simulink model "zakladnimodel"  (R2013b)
settings: Solver=FixedStepDiscrete  StartTime=0.0  StopTime=132.0  FixedStep=1  RelTol=1e-3

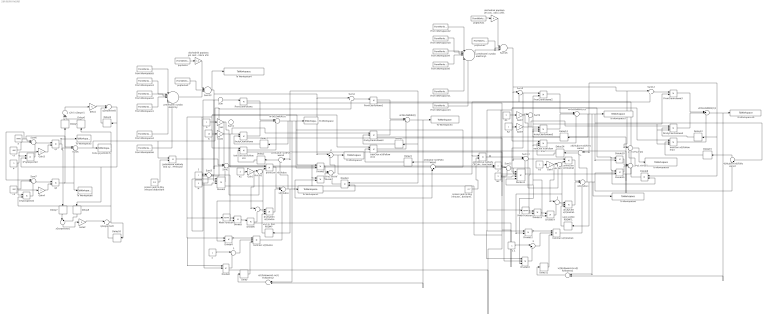
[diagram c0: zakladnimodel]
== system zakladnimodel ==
  " " : Sum  Inputs=|++
  " x1(t-1) POC PODM?" : Delay  DelayLength=1  InitialCondition=0
  " x1(t-1) POC PODM?1" : Delay  DelayLength=1  InitialCondition=0
  " x(t)Followera1+x(t)Followera1" : Sum  Inputs=|++
  " x(t)Followera1+x(t)Followera2" : Sum  Inputs=|++
   x(t)Vudce+x(t)Followera{1..4} (4 alike) : Sum  Inputs=|++
  " x2t-1-x2expt-1" : Sum  Inputs=|+-
  " 1" : Sum  Inputs=|+-
  " 2" : Sum  Inputs=|++
  " 2A+2K1" : Sum  Inputs=|++
  " 2A+2K2" : Sum  Inputs=|++
  " 3" : Sum  Inputs=|+-
  " A*x1+A*xV" : Sum  Inputs=|+++
  " A*x1+A*xV1" : Sum  Inputs=|+++
  " P" : Sum  Inputs=|+-
  " prednostni vyroba elektriny" : Sum  Inputs=|+++++++
  " prednostni vyroba elektriny1" : Sum  Inputs=|+++++++
  " q1expectedt" : Sum  Inputs=|++
  " q2expectedt " : Sum  Inputs=|++
  " x(t)Vudce" : Sum  Inputs=|++-
  " x(t)Vudce1" : Sum  Inputs=|++-
  " x2expectedt1" : Sum  Inputs=|+-
  " xFOLLOWER1(t)" : Sum  Inputs=|++-
  " xFOLLOWER1(t)1" : Sum  Inputs=|++-
  " xFOLLOWER2(t)" : Sum  Inputs=|++-
  " xFOLLOWER2(t)1" : Sum  Inputs=|++-
  1 : Constant
  "1 " : Constant
  1 1 : Constant
  2 : Constant
  A : Constant
  A1 : Constant
  "Cena je jednotk.N " : ToWorkspace  VariableName=Puhli  SampleTime=-1  SaveFormat=Timeseries
  Delay{,1..15} (16 alike) : Delay  DelayLength=1  InitialCondition=0
  Divide{1..2,5,7,9..10,13,15} (8 alike) : Product  Inputs=**
  Divide11 : Product  Inputs=***/
  Divide{4,6,12,14} (4 alike) : Product  Inputs=*/
  Divide16 : Product  Inputs=**/
  Divide3 : Product  Inputs=***/
  Divide8 : Product  Inputs=**/
  DruhyClenFollowa{,1..3} (4 alike) : Product  Inputs=**/
  From Workspace1 : FromWorkspace  VariableName=FVE  SampleTime=0
  From Workspace10 : FromWorkspace  VariableName=JE  SampleTime=0
  From Workspace11 : FromWorkspace  VariableName=ostatni  SampleTime=0
  From Workspace12 : FromWorkspace  VariableName=bioplyn  SampleTime=0
  From Workspace13 : FromWorkspace  VariableName=biomasa  SampleTime=0
  From Workspace2 : FromWorkspace  VariableName=VE  SampleTime=0
  From Workspace3 : FromWorkspace  VariableName=JE  SampleTime=0
  From Workspace4 : FromWorkspace  VariableName=ostatni  SampleTime=0
  From Workspace5 : FromWorkspace  VariableName=bioplyn  SampleTime=0
  From Workspace6 : FromWorkspace  VariableName=biomasa  SampleTime=0
  From Workspace8 : FromWorkspace  VariableName=FVE  SampleTime=0
  From Workspace9 : FromWorkspace  VariableName=VE  SampleTime=0
  Gain{,1..7} (8 alike) : Gain  Gain=2
  K : Constant  Value=10
  K1 : Constant  Value=2
  K2 : Constant
  K3 : Constant
  Math Function : Math  Operator=square
  Math Function1 : Math  Operator=square
  N : Constant  Value=3
  N1 : Constant  Value=3
  PrvniClenFollowa{,1..3} (4 alike) : Product  Inputs=*/
  Sum{,4,8,12} (4 alike) : Sum  Inputs=|+-
  Sum1 : Sum  Inputs=|++
  Sum10 : Sum  Inputs=|-+-
  Sum11 : Sum  Inputs=|-+
  Sum13 : Sum  Inputs=|++--
  Sum15 : Sum  Inputs=|++-
  Sum2 : Sum  Inputs=|-+-
  Sum3 : Sum  Inputs=|-+
  Sum5 : Sum  Inputs=|+--
  Sum6 : Sum  Inputs=|+--
  Sum7 : Sum  Inputs=|+--
  Sum9 : Sum  Inputs=|++
  To Workspace : ToWorkspace  VariableName=qFolloweraVyrobceUhli1  SampleTime=-1  SaveFormat=Timeseries
  To Workspace1 : ToWorkspace  VariableName=qVudceVyrobceUhli  SampleTime=-1  SaveFormat=Timeseries
  To Workspace10 : ToWorkspace  VariableName=qFolloweraObchodnika2  SampleTime=-1  SaveFormat=Timeseries
  To Workspace2 : ToWorkspace  VariableName=PelektrinyZuhli  SampleTime=-1  SaveFormat=Timeseries
  To Workspace3 : ToWorkspace  VariableName=qFolloweraVyrobceUhli2  SampleTime=-1  SaveFormat=Timeseries
  To Workspace4 : ToWorkspace  VariableName=poptavkaUvyrobcuElzUhli  SampleTime=-1  SaveFormat=Timeseries
  To Workspace5 : ToWorkspace  VariableName=q1uhli  SampleTime=-1  SaveFormat=Timeseries
  To Workspace6 : ToWorkspace  VariableName=q2uhli  SampleTime=-1  SaveFormat=Timeseries
  To Workspace7 : ToWorkspace  VariableName=qFolloweraObchodnika1  SampleTime=-1  SaveFormat=Timeseries
  To Workspace8 : ToWorkspace  VariableName=qVudceObchodnika  SampleTime=-1  SaveFormat=Timeseries
  To Workspace9 : ToWorkspace  VariableName=PmaloobchodniObchodniku  SampleTime=-1  SaveFormat=Timeseries
  "a " : Constant  Value=6000
  "b " : Constant
  b*q1expected : Product
  b*q2expected : Product
  beta1 : Gain
  beta2 : Gain
  c1 : Constant  Value=400
  c2 : Constant  Value=400
  druhyClen x(t)Vudce : Product  Inputs=*/*
  druhyClen x(t)Vudce1 : Product  Inputs=*/*
  "jednotkove naklady ČEZ obchodníka který má mít dominant.pozici 44% trzni podil " : Product  Inputs=**
  jednotkove naklady ČEZ výrobce P-Pinhouse : Product  Inputs=**
  obchodnik poptava jen cast od vyrobcu uhli : Gain  Gain=1.2
  obchodnik poptava jen cast od vyrobcu uhli1 : Gain
  p=b-a*sumaQ : Sum  Inputs=|+-
  poptavka : FromWorkspace  VariableName=nettospotreba  SampleTime=0
  poptavka1 : FromWorkspace  VariableName=nettospotreba  SampleTime=0
  poptavka2 : FromWorkspace  VariableName=vyvoz  SampleTime=0
  poptavka3 : FromWorkspace  VariableName=vyvoz  SampleTime=0
  prvniClen x(t)Vudce : Product  Inputs=*/
  prvniClen x(t)Vudce1 : Product  Inputs=*/
  q1 : Product  Inputs=*/
  q2 : Product  Inputs=*/
  snizeni jedn N diky inhouse dodavkam : Constant  Value=0.8
  "snizeni jedn N diky inhouse dodavkam1 " : Constant  Value=0.7
  tretiClen x(t)Followera{,1..3} (4 alike) : Product  Inputs=**/
  tretiClen x(t)Vudce : Product  Inputs=***
  tretiClen x(t)Vudce1 : Product  Inputs=***
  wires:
  Sum13/1 -> To Workspace4/1, Sum2/2, Sum/1, Sum4/1, " P"/1
  Sum/1 -> Divide3/1, PrvniClenFollowa/1
  Gain/1 -> " 2A+2K1"/2, Sum1/1
  K/1 -> Gain1/1
  PrvniClenFollowa/1 -> " xFOLLOWER1(t)"/1
  DruhyClenFollowa/1 -> " xFOLLOWER1(t)"/2
  tretiClen x(t)Followera/1 -> " xFOLLOWER1(t)"/3
  N/1 -> Sum3/2, Divide8/2
  1/1 -> Sum3/1
  Sum3/1 -> Divide5/1, Divide3/2
  Divide3/1 -> Sum2/3
  Sum2/1 -> prvniClen x(t)Vudce/1
  K1/1 -> Gain2/1
  Gain2/1 -> " "/1, " 2A+2K1"/1
  " 2A+2K1"/1 -> prvniClen x(t)Vudce/2, Divide4/2, druhyClen x(t)Vudce/2
  " "/1 -> druhyClen x(t)Vudce/1
  Math Function/1 -> Divide5/2
  Divide6/1 -> " "/2
  Divide5/1 -> Divide6/1
  "1 "/1 -> " 1"/1
  Divide4/1 -> tretiClen x(t)Vudce/1
  " 1"/1 -> tretiClen x(t)Vudce/2
  Divide8/1 -> " 1"/2
  Delay/1 -> tretiClen x(t)Vudce/3
  prvniClen x(t)Vudce/1 -> " x(t)Vudce"/1
  druhyClen x(t)Vudce/1 -> " x(t)Vudce"/2
  tretiClen x(t)Vudce/1 -> " x(t)Vudce"/3
  " x(t)Vudce"/1 -> " x(t)Vudce+x(t)Followera2"/2, " x(t)Vudce+x(t)Followera1"/1, Divide7/2, To Workspace1/1, " x1(t-1) POC PODM?"/1
  " x1(t-1) POC PODM?"/1 -> druhyClen x(t)Vudce/3
  Divide2/1 -> " A*x1+A*xV"/1
  Divide7/1 -> " A*x1+A*xV"/2
  " A*x1+A*xV"/1 -> " P"/2
  Sum4/1 -> PrvniClenFollowa1/1
  Gain1/1 -> DruhyClenFollowa1/1, DruhyClenFollowa/1, Sum1/2
  A/1 -> tretiClen x(t)Followera1/1, Divide1/2, Divide7/1, Divide2/1, Divide8/1, Divide4/1, Math Function/1, Divide3/3, tretiClen x(t)Followera/1, Gain/1
  Sum1/1 -> tretiClen x(t)Followera1/3, DruhyClenFollowa1/3, PrvniClenFollowa1/2, Divide8/3, Divide3/4, Divide6/2, tretiClen x(t)Followera/3, DruhyClenFollowa/3, PrvniClenFollowa/2
  PrvniClenFollowa1/1 -> " xFOLLOWER2(t)"/1
  DruhyClenFollowa1/1 -> " xFOLLOWER2(t)"/2
  tretiClen x(t)Followera1/1 -> " xFOLLOWER2(t)"/3
  " xFOLLOWER2(t)"/1 -> " x(t)Vudce+x(t)Followera2"/1, Delay2/1, Divide1/1, To Workspace3/1, " x(t)Followera1+x(t)Followera2"/2
  " x(t)Followera1+x(t)Followera2"/1 -> Delay/1
  Divide1/1 -> " A*x1+A*xV"/3
  " xFOLLOWER1(t)"/1 -> Delay1/1, Divide2/2, " x(t)Vudce+x(t)Followera1"/2, To Workspace/1, " x(t)Followera1+x(t)Followera2"/1
  Delay1/1 -> DruhyClenFollowa/2
  Delay2/1 -> DruhyClenFollowa1/2
  " x(t)Vudce+x(t)Followera2"/1 -> Delay3/1
  Delay3/1 -> tretiClen x(t)Followera/2
  " x(t)Vudce+x(t)Followera1"/1 -> Delay4/1
  Delay4/1 -> tretiClen x(t)Followera1/2
  "a "/1 -> Sum7/1, Sum5/1, Sum6/1
  c1/1 -> Sum6/2
  "b "/1 -> Gain4/1, b*q1expected/1, Gain3/1, b*q2expected/1
  b*q2expected/1 -> Sum6/3
  Sum6/1 -> q1/1
  Gain3/1 -> q1/2
  c2/1 -> Sum7/2
  b*q1expected/1 -> Sum7/3
  Sum7/1 -> q2/1
  Gain4/1 -> q2/2
  q1/1 -> To Workspace5/1, Delay7/1, Sum5/2
  q2/1 -> To Workspace6/1, Sum5/3, Delay5/1
  " q2expectedt "/1 -> Delay9/1, Delay8/1, b*q2expected/2
  " x2expectedt1"/1 -> beta2/1
  " x2t-1-x2expt-1"/1 -> beta1/1
  Delay5/1 -> " x2t-1-x2expt-1"/1
  " q1expectedt"/1 -> Delay10/1, b*q1expected/2, Delay6/1
  Delay6/1 -> " x2t-1-x2expt-1"/2
  beta1/1 -> " q2expectedt "/1
  Delay7/1 -> " x2expectedt1"/1
  Delay8/1 -> " x2expectedt1"/2
  beta2/1 -> " q1expectedt"/1
  Delay9/1 -> " q2expectedt "/2
  Delay10/1 -> " q1expectedt"/2
  Sum15/1 -> Sum12/1, p=b-a*sumaQ/1, Sum10/2, Sum8/1
  Sum8/1 -> Divide11/1, PrvniClenFollowa2/1
  Gain5/1 -> " 2A+2K2"/2, Sum9/1
  K2/1 -> Gain6/1
  PrvniClenFollowa2/1 -> " xFOLLOWER1(t)1"/1
  DruhyClenFollowa2/1 -> " xFOLLOWER1(t)1"/2
  tretiClen x(t)Followera2/1 -> " xFOLLOWER1(t)1"/3
  N1/1 -> Sum11/2, Divide16/2
  2/1 -> Sum11/1
  Sum11/1 -> Divide13/1, Divide11/2
  Divide11/1 -> Sum10/3
  Sum10/1 -> prvniClen x(t)Vudce1/1
  K3/1 -> Gain7/1
  Gain7/1 -> " 2"/1, " 2A+2K2"/1
  " 2A+2K2"/1 -> prvniClen x(t)Vudce1/2, Divide12/2, druhyClen x(t)Vudce1/2
  " 2"/1 -> druhyClen x(t)Vudce1/1
  Math Function1/1 -> Divide13/2
  Divide14/1 -> " 2"/2
  Divide13/1 -> Divide14/1
  1 1/1 -> " 3"/1
  Divide12/1 -> tretiClen x(t)Vudce1/1
  " 3"/1 -> tretiClen x(t)Vudce1/2
  Divide16/1 -> " 3"/2
  Delay11/1 -> tretiClen x(t)Vudce1/3
  prvniClen x(t)Vudce1/1 -> " x(t)Vudce1"/1
  druhyClen x(t)Vudce1/1 -> " x(t)Vudce1"/2
  tretiClen x(t)Vudce1/1 -> " x(t)Vudce1"/3
  " x(t)Vudce1"/1 -> " x(t)Vudce+x(t)Followera4"/2, " x(t)Vudce+x(t)Followera3"/1, Divide15/2, To Workspace8/1, " x1(t-1) POC PODM?1"/1
  " x1(t-1) POC PODM?1"/1 -> druhyClen x(t)Vudce1/3
  Divide10/1 -> " A*x1+A*xV1"/1
  Divide15/1 -> " A*x1+A*xV1"/2
  " A*x1+A*xV1"/1 -> p=b-a*sumaQ/2
  p=b-a*sumaQ/1 -> To Workspace9/1
  Sum12/1 -> PrvniClenFollowa3/1
  Gain6/1 -> DruhyClenFollowa3/1, DruhyClenFollowa2/1, Sum9/2
  A1/1 -> tretiClen x(t)Followera3/1, Divide9/2, Divide15/1, Divide10/1, Divide16/1, Divide12/1, Math Function1/1, Divide11/3, tretiClen x(t)Followera2/1, Gain5/1
  Sum9/1 -> tretiClen x(t)Followera3/3, DruhyClenFollowa3/3, PrvniClenFollowa3/2, Divide16/3, Divide11/4, Divide14/2, tretiClen x(t)Followera2/3, DruhyClenFollowa2/3, PrvniClenFollowa2/2
  PrvniClenFollowa3/1 -> " xFOLLOWER2(t)1"/1
  DruhyClenFollowa3/1 -> " xFOLLOWER2(t)1"/2
  tretiClen x(t)Followera3/1 -> " xFOLLOWER2(t)1"/3
  " xFOLLOWER2(t)1"/1 -> " x(t)Vudce+x(t)Followera4"/1, Delay13/1, Divide9/1, To Workspace10/1, " x(t)Followera1+x(t)Followera1"/2
  " x(t)Followera1+x(t)Followera1"/1 -> Delay11/1
  Divide9/1 -> " A*x1+A*xV1"/3
  " xFOLLOWER1(t)1"/1 -> Delay12/1, Divide10/2, " x(t)Vudce+x(t)Followera3"/2, To Workspace7/1, " x(t)Followera1+x(t)Followera1"/1
  Delay12/1 -> DruhyClenFollowa2/2
  Delay13/1 -> DruhyClenFollowa3/2
  " x(t)Vudce+x(t)Followera4"/1 -> Delay14/1
  Delay14/1 -> tretiClen x(t)Followera2/2
  " x(t)Vudce+x(t)Followera3"/1 -> Delay15/1
  Delay15/1 -> tretiClen x(t)Followera3/2
  snizeni jedn N diky inhouse dodavkam/1 -> jednotkove naklady ČEZ výrobce P-Pinhouse/2
  From Workspace5/1 -> " prednostni vyroba elektriny"/1
  From Workspace3/1 -> " prednostni vyroba elektriny"/2
  From Workspace2/1 -> " prednostni vyroba elektriny"/3
  Sum5/1 -> jednotkove naklady ČEZ výrobce P-Pinhouse/1, Sum4/2, Sum/2, "Cena je jednotk.N "/1
  From Workspace1/1 -> " prednostni vyroba elektriny"/4
  From Workspace4/1 -> " prednostni vyroba elektriny"/6
  From Workspace6/1 -> " prednostni vyroba elektriny"/7
  poptavka/1 -> obchodnik poptava jen cast od vyrobcu uhli/1
  obchodnik poptava jen cast od vyrobcu uhli/1 -> Sum13/1
  " prednostni vyroba elektriny"/1 -> Sum13/3
  From Workspace12/1 -> " prednostni vyroba elektriny1"/1
  From Workspace10/1 -> " prednostni vyroba elektriny1"/2
  From Workspace9/1 -> " prednostni vyroba elektriny1"/3
  From Workspace8/1 -> " prednostni vyroba elektriny1"/4
  From Workspace11/1 -> " prednostni vyroba elektriny1"/6
  From Workspace13/1 -> " prednostni vyroba elektriny1"/7
  poptavka1/1 -> obchodnik poptava jen cast od vyrobcu uhli1/1
  obchodnik poptava jen cast od vyrobcu uhli1/1 -> Sum15/1
  jednotkove naklady ČEZ výrobce P-Pinhouse/1 -> Sum2/1
  "snizeni jedn N diky inhouse dodavkam1 "/1 -> "jednotkove naklady ČEZ obchodníka který má mít dominant.pozici 44% trzni podil "/2
  " P"/1 -> "jednotkove naklady ČEZ obchodníka který má mít dominant.pozici 44% trzni podil "/1, Sum8/2, Sum12/2, To Workspace2/1
  "jednotkove naklady ČEZ obchodníka který má mít dominant.pozici 44% trzni podil "/1 -> Sum10/1
  " prednostni vyroba elektriny1"/1 -> Sum15/3
  poptavka2/1 -> Sum15/2
  poptavka3/1 -> Sum13/2
